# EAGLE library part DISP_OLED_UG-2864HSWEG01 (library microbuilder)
UG-2864HSWEG01 OLED display Both 1.3" and 0.96" models share the same FPC tab footprint, only the screen dimensions vary.
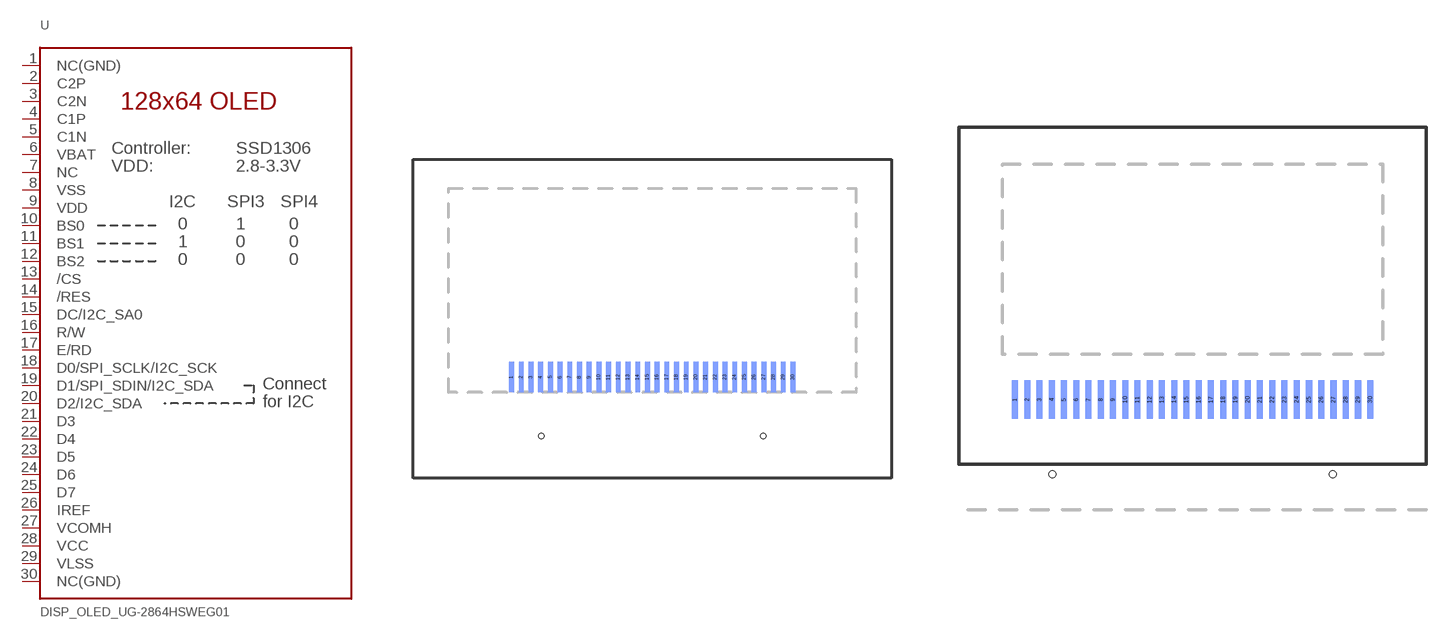
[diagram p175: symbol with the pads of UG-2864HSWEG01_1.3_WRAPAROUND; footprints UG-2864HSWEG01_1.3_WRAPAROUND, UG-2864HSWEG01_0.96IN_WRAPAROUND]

Designator prefix U

## DISP_OLED_UG-2864HSWEG01  [UG-2864HSWEG01_1.3_WRAPAROUND]
1  NC(GND)  in
2  C2P  in
3  C2N  in
4  C1P  in
5  C1N  in
6  VBAT  in
7  NC  nc
8  VSS  pwr
9  VDD  pwr
10  BS0  in
11  BS1  in
12  BS2  in
13  /CS  in
14  /RES  in
15  DC/I2C_SA0  in
16  R/W  in
17  E/RD  in
18  D0/SPI_SCLK/I2C_SCK
19  D1/SPI_SDIN/I2C_SDA
20  D2/I2C_SDA
21  D3
22  D4
23  D5
24  D6
25  D7
26  IREF  in
27  VCOMH  out
28  VCC  pwr
29  VLSS  pwr
30  NC(GND)  in

## DISP_OLED_UG-2864HSWEG010.96"  [UG-2864HSWEG01_0.96IN_WRAPAROUND]
Pads as for UG-2864HSWEG01_1.3_WRAPAROUND

## Footprint UG-2864HSWEG01_1.3_WRAPAROUND (pad centres in mm)
smd 0.35 x 2.2 bottom: 1 -10.15,-0.2; 2 -9.45,-0.2; 3 -8.75,-0.2; 4 -8.05,-0.2; 5 -7.35,-0.2; 6 -6.65,-0.2; 7 -5.95,-0.2; 8 -5.25,-0.2; 9 -4.55,-0.2; 10 -3.85,-0.2; 11 -3.15,-0.2; 12 -2.45,-0.2; 13 -1.75,-0.2; 14 -1.05,-0.2; 15 -0.35,-0.2; 16 0.35,-0.2; 17 1.05,-0.2; 18 1.75,-0.2; 19 2.45,-0.2; 20 3.15,-0.2; 21 3.85,-0.2; 22 4.55,-0.2; 23 5.25,-0.2; 24 5.95,-0.2; 25 6.65,-0.2; 26 7.35,-0.2; 27 8.05,-0.2; 28 8.75,-0.2; 29 9.45,-0.2; 30 10.15,-0.2
hole 0.4 at -8,-4.45
hole 0.4 at 8,-4.45

## Footprint UG-2864HSWEG01_0.96IN_WRAPAROUND (pad centres in mm)
smd 0.35 x 2.2 bottom: 1 -10.15,-1.2; 2 -9.45,-1.2; 3 -8.75,-1.2; 4 -8.05,-1.2; 5 -7.35,-1.2; 6 -6.65,-1.2; 7 -5.95,-1.2; 8 -5.25,-1.2; 9 -4.55,-1.2; 10 -3.85,-1.2; 11 -3.15,-1.2; 12 -2.45,-1.2; 13 -1.75,-1.2; 14 -1.05,-1.2; 15 -0.35,-1.2; 16 0.35,-1.2; 17 1.05,-1.2; 18 1.75,-1.2; 19 2.45,-1.2; 20 3.15,-1.2; 21 3.85,-1.2; 22 4.55,-1.2; 23 5.25,-1.2; 24 5.95,-1.2; 25 6.65,-1.2; 26 7.35,-1.2; 27 8.05,-1.2; 28 8.75,-1.2; 29 9.45,-1.2; 30 10.15,-1.2
hole 0.4 at -8,-5.45
hole 0.4 at 8,-5.45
